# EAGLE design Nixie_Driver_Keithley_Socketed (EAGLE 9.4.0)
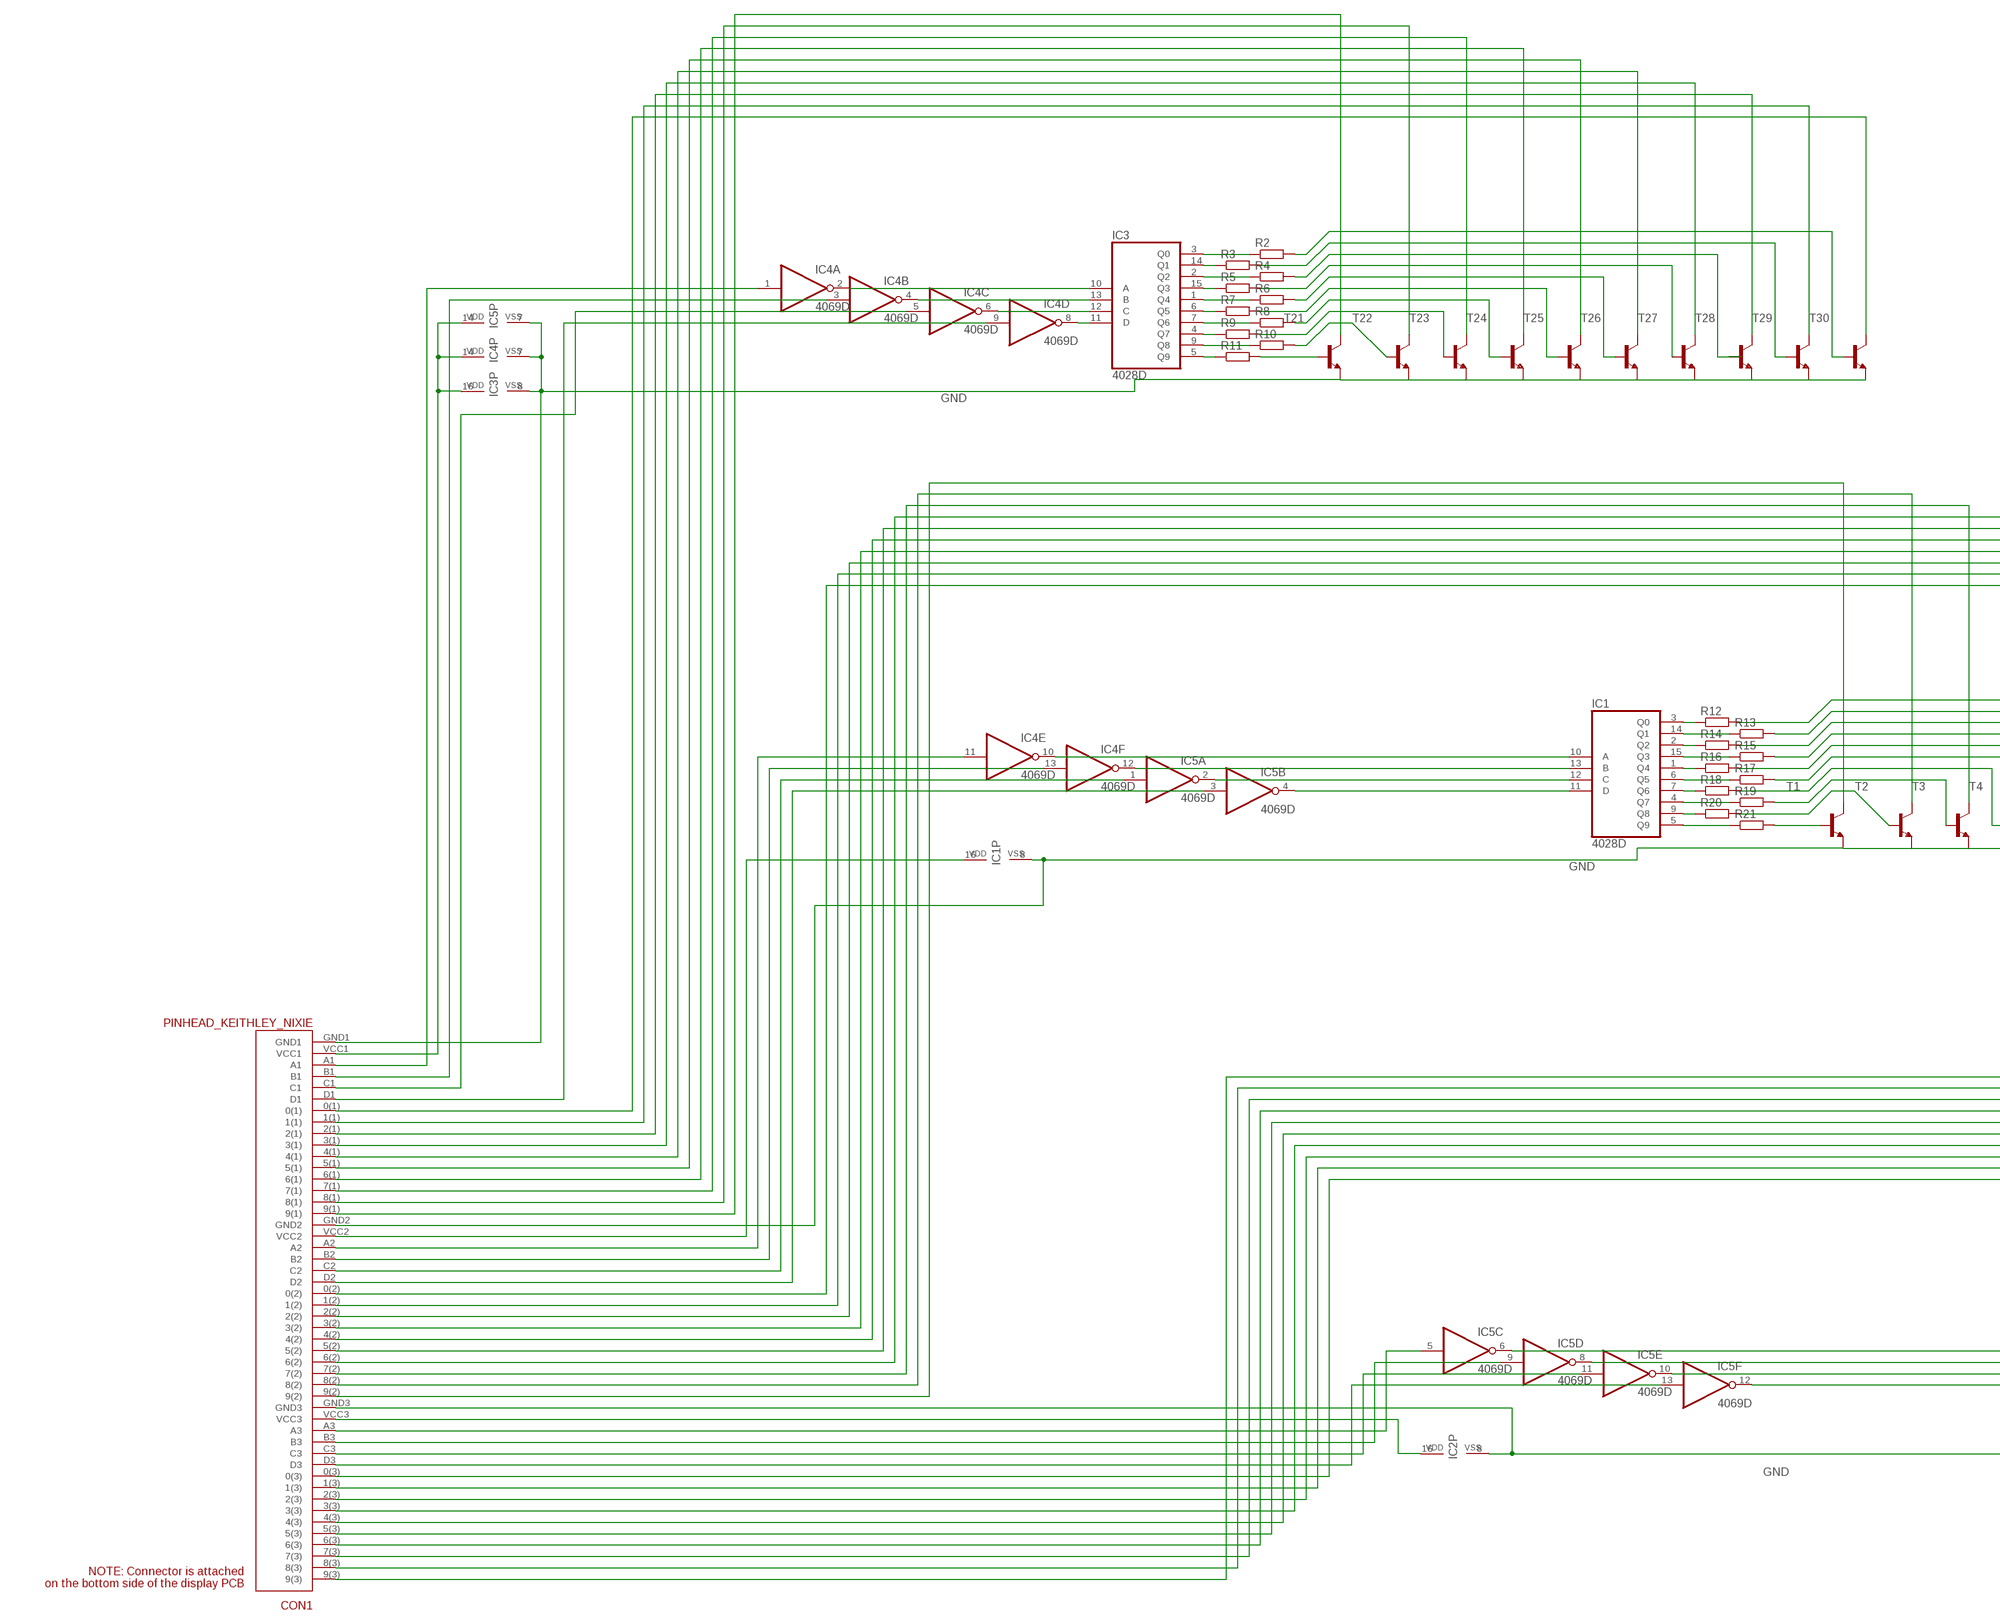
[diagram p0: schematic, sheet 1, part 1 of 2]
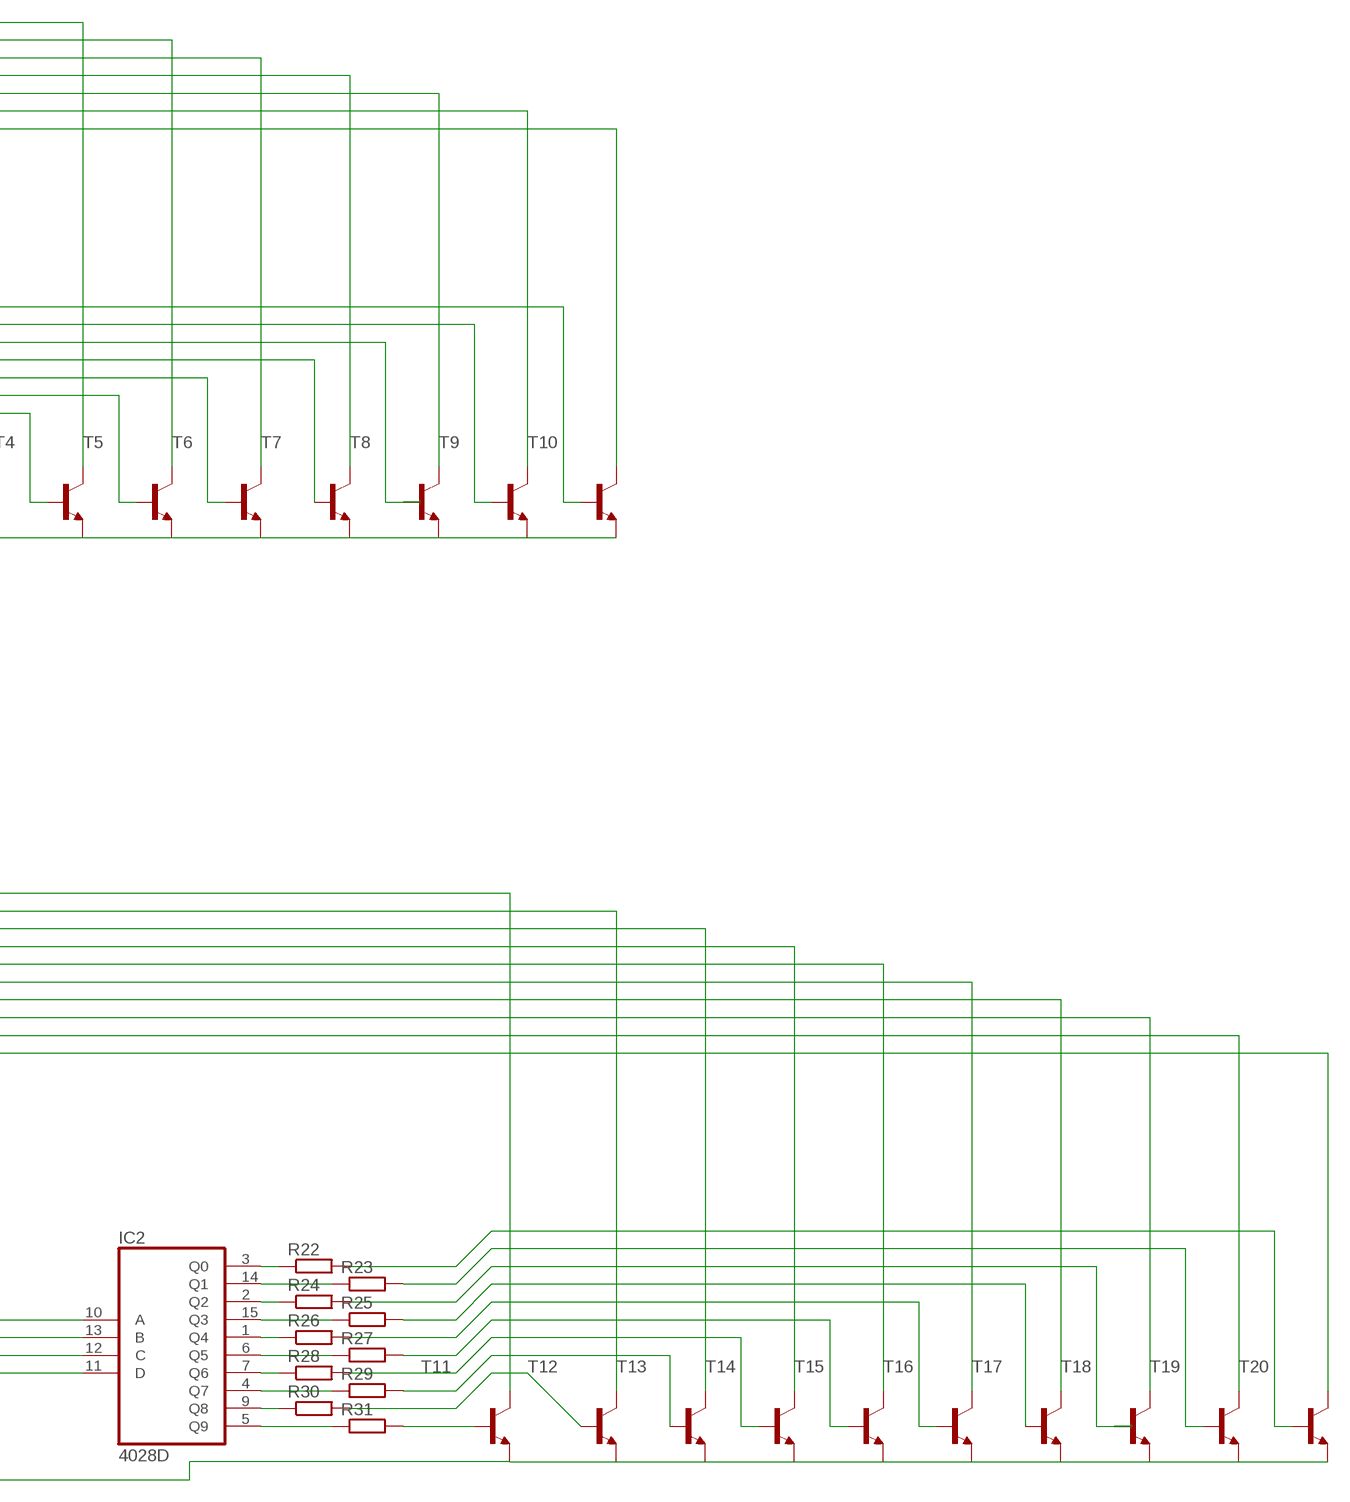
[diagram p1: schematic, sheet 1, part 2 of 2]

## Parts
CON1  PINHEAD_KEITHLEY_NIXIE  [PINHEAD_KEITHLEY_NIXIE]
IC1  4028D  [SO16]
IC2  4028D  [SO16]
IC3  4028D  [SO16]
IC4  4069D  [SO14]
IC5  4069D  [SO14]
R2  R-EU_R0402  [R0402]
R3  R-EU_R0402  [R0402]
R4  R-EU_R0402  [R0402]
R5  R-EU_R0402  [R0402]
R6  R-EU_R0402  [R0402]
R7  R-EU_R0402  [R0402]
R8  R-EU_R0402  [R0402]
R9  R-EU_R0402  [R0402]
R10  R-EU_R0402  [R0402]
R11  R-EU_R0402  [R0402]
R12  R-EU_R0402  [R0402]
R13  R-EU_R0402  [R0402]
R14  R-EU_R0402  [R0402]
R15  R-EU_R0402  [R0402]
R16  R-EU_R0402  [R0402]
R17  R-EU_R0402  [R0402]
R18  R-EU_R0402  [R0402]
R19  R-EU_R0402  [R0402]
R20  R-EU_R0402  [R0402]
R21  R-EU_R0402  [R0402]
R22  R-EU_R0402  [R0402]
R23  R-EU_R0402  [R0402]
R24  R-EU_R0402  [R0402]
R25  R-EU_R0402  [R0402]
R26  R-EU_R0402  [R0402]
R27  R-EU_R0402  [R0402]
R28  R-EU_R0402  [R0402]
R29  R-EU_R0402  [R0402]
R30  R-EU_R0402  [R0402]
R31  R-EU_R0402  [R0402]
T1  MMBTA42LT1-NPN-SOT23-BEC  [SOT23-BEC]
T2  MMBTA42LT1-NPN-SOT23-BEC  [SOT23-BEC]
T3  MMBTA42LT1-NPN-SOT23-BEC  [SOT23-BEC]
T4  MMBTA42LT1-NPN-SOT23-BEC  [SOT23-BEC]
T5  MMBTA42LT1-NPN-SOT23-BEC  [SOT23-BEC]
T6  MMBTA42LT1-NPN-SOT23-BEC  [SOT23-BEC]
T7  MMBTA42LT1-NPN-SOT23-BEC  [SOT23-BEC]
T8  MMBTA42LT1-NPN-SOT23-BEC  [SOT23-BEC]
T9  MMBTA42LT1-NPN-SOT23-BEC  [SOT23-BEC]
T10  MMBTA42LT1-NPN-SOT23-BEC  [SOT23-BEC]
T11  MMBTA42LT1-NPN-SOT23-BEC  [SOT23-BEC]
T12  MMBTA42LT1-NPN-SOT23-BEC  [SOT23-BEC]
T13  MMBTA42LT1-NPN-SOT23-BEC  [SOT23-BEC]
T14  MMBTA42LT1-NPN-SOT23-BEC  [SOT23-BEC]
T15  MMBTA42LT1-NPN-SOT23-BEC  [SOT23-BEC]
T16  MMBTA42LT1-NPN-SOT23-BEC  [SOT23-BEC]
T17  MMBTA42LT1-NPN-SOT23-BEC  [SOT23-BEC]
T18  MMBTA42LT1-NPN-SOT23-BEC  [SOT23-BEC]
T19  MMBTA42LT1-NPN-SOT23-BEC  [SOT23-BEC]
T20  MMBTA42LT1-NPN-SOT23-BEC  [SOT23-BEC]
T21  MMBTA42LT1-NPN-SOT23-BEC  [SOT23-BEC]
T22  MMBTA42LT1-NPN-SOT23-BEC  [SOT23-BEC]
T23  MMBTA42LT1-NPN-SOT23-BEC  [SOT23-BEC]
T24  MMBTA42LT1-NPN-SOT23-BEC  [SOT23-BEC]
T25  MMBTA42LT1-NPN-SOT23-BEC  [SOT23-BEC]
T26  MMBTA42LT1-NPN-SOT23-BEC  [SOT23-BEC]
T27  MMBTA42LT1-NPN-SOT23-BEC  [SOT23-BEC]
T28  MMBTA42LT1-NPN-SOT23-BEC  [SOT23-BEC]
T29  MMBTA42LT1-NPN-SOT23-BEC  [SOT23-BEC]
T30  MMBTA42LT1-NPN-SOT23-BEC  [SOT23-BEC]

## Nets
GND: CON1.GND1 CON1.GND2 CON1.GND3 IC1.8(VSS) IC2.8(VSS) IC3.8(VSS) IC4.7(P:VSS) IC5.7(P:VSS) T1.E T2.E T3.E T4.E T5.E T6.E T7.E T8.E T9.E T10.E T11.E T12.E T13.E T14.E T15.E T16.E T17.E T18.E T19.E T20.E T21.E T22.E T23.E T24.E T25.E T26.E T27.E T28.E T29.E T30.E
N$1: IC1.5(Q9) R21.1
N$2: R20.2 T2.B
N$3: R19.2 T3.B
N$4: R18.2 T4.B
N$5: R17.2 T5.B
N$6: R16.2 T6.B
N$7: R15.2 T7.B
N$8: R14.2 T8.B
N$9: R13.2 T9.B
N$10: R12.2 T10.B
N$11: IC3.10(A) IC4.2(A:O)
N$12 [HV_Cathodes]: CON1.9(2) T1.C
N$13 [HV_Cathodes]: CON1.7(2) T3.C
N$14 [HV_Cathodes]: CON1.5(2) T5.C
N$15 [HV_Cathodes]: CON1.3(2) T7.C
N$16 [HV_Cathodes]: CON1.1(2) T9.C
N$17 [HV_Cathodes]: CON1.8(2) T2.C
N$18: CON1.A2 IC4.11(E:I)
N$19 [HV_Cathodes]: CON1.0(2) T10.C
N$20 [HV_Cathodes]: CON1.2(2) T8.C
N$21 [HV_Cathodes]: CON1.4(2) T6.C
N$22 [HV_Cathodes]: CON1.6(2) T4.C
N$23 [HV_Cathodes]: CON1.8(1) T22.C
N$24: CON1.B2 IC4.13(F:I)
N$25: CON1.VCC2 IC1.16(VDD)
N$26: CON1.C2 IC5.1(A:I)
N$27 [HV_Cathodes]: CON1.8(3) T12.C
N$28: R31.2 T11.B
N$29: R30.2 T12.B
N$30: R29.2 T13.B
N$31: R28.2 T14.B
N$32: R27.2 T15.B
N$33: R26.2 T16.B
N$34: R25.2 T17.B
N$35: R24.2 T18.B
N$36: R23.2 T19.B
N$37: R22.2 T20.B
N$38: IC3.13(B) IC4.4(B:O)
N$39 [HV_Cathodes]: CON1.9(3) T11.C
N$40 [HV_Cathodes]: CON1.7(3) T13.C
N$41 [HV_Cathodes]: CON1.5(3) T15.C
N$42 [HV_Cathodes]: CON1.3(3) T17.C
N$43 [HV_Cathodes]: CON1.1(3) T19.C
N$44: CON1.D2 IC5.3(B:I)
N$45: CON1.A3 IC5.5(C:I)
N$46 [HV_Cathodes]: CON1.0(3) T20.C
N$47 [HV_Cathodes]: CON1.2(3) T18.C
N$48 [HV_Cathodes]: CON1.4(3) T16.C
N$49 [HV_Cathodes]: CON1.6(3) T14.C
N$50: IC3.12(C) IC4.6(C:O)
N$51: CON1.B3 IC5.9(D:I)
N$52: CON1.VCC3 IC2.16(VDD)
N$53: CON1.VCC1 IC3.16(VDD) IC4.14(P:VDD) IC5.14(P:VDD)
N$54: CON1.C3 IC5.11(E:I)
N$55: IC3.11(D) IC4.8(D:O)
N$56: CON1.C1 IC4.5(C:I)
N$57: CON1.D3 IC5.13(F:I)
N$58: IC1.10(A) IC4.10(E:O)
N$59: IC1.13(B) IC4.12(F:O)
N$60: IC1.12(C) IC5.2(A:O)
N$61: IC1.11(D) IC5.4(B:O)
N$62: IC2.10(A) IC5.6(C:O)
N$63: IC2.13(B) IC5.8(D:O)
N$64: IC2.12(C) IC5.10(E:O)
N$65: IC2.11(D) IC5.12(F:O)
N$66: IC3.3(Q0) R2.1
N$67: IC3.14(Q1) R3.1
N$68: IC3.2(Q2) R4.1
N$69: IC3.15(Q3) R5.1
N$70: IC3.1(Q4) R6.1
N$71: IC3.6(Q5) R7.1
N$72: IC3.7(Q6) R8.1
N$73: IC3.4(Q7) R9.1
N$74: IC3.9(Q8) R10.1
N$75: IC3.5(Q9) R11.1
N$76: IC1.3(Q0) R12.1
N$77: IC1.14(Q1) R13.1
N$78: IC1.2(Q2) R14.1
N$79: IC1.15(Q3) R15.1
N$80: IC1.1(Q4) R16.1
N$81: IC1.6(Q5) R17.1
N$82: IC1.7(Q6) R18.1
N$83: IC1.4(Q7) R19.1
N$84: IC1.9(Q8) R20.1
N$85: R11.2 T21.B
N$86: R10.2 T22.B
N$87: R9.2 T23.B
N$88: R8.2 T24.B
N$89: R7.2 T25.B
N$90: R6.2 T26.B
N$91: R5.2 T27.B
N$92: R4.2 T28.B
N$93: R3.2 T29.B
N$94: R2.2 T30.B
N$95: R21.2 T1.B
N$96 [HV_Cathodes]: CON1.9(1) T21.C
N$97 [HV_Cathodes]: CON1.7(1) T23.C
N$98 [HV_Cathodes]: CON1.5(1) T25.C
N$99 [HV_Cathodes]: CON1.3(1) T27.C
N$100 [HV_Cathodes]: CON1.1(1) T29.C
N$101: CON1.A1 IC4.1(A:I)
N$102: CON1.B1 IC4.3(B:I)
N$103: IC2.3(Q0) R22.1
N$104 [HV_Cathodes]: CON1.0(1) T30.C
N$105 [HV_Cathodes]: CON1.2(1) T28.C
N$106 [HV_Cathodes]: CON1.4(1) T26.C
N$107 [HV_Cathodes]: CON1.6(1) T24.C
N$108: IC2.14(Q1) R23.1
N$109: CON1.D1 IC4.9(D:I)
N$110: IC2.2(Q2) R24.1
N$111: IC2.15(Q3) R25.1
N$112: IC2.1(Q4) R26.1
N$113: IC2.6(Q5) R27.1
N$114: IC2.7(Q6) R28.1
N$115: IC2.4(Q7) R29.1
N$116: IC2.9(Q8) R30.1
N$117: IC2.5(Q9) R31.1

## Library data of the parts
CON1 = DIL_Style_Pinhead_Connectors:PINHEAD_KEITHLEY_NIXIE
IC1-IC3 = 40xx:4028: BCD to decimal DECODER
IC4 IC5 = 40xx:4069: Hex INVERTER
R2-R31 = rcl:R-EU_: RESISTOR, European symbol; SPICEPREFIX: R
T1-T30 = transistor-neu-to92:*-NPN-: NPN Transistror

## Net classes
0 LV_Signal: width 0.25 mm, clearance 0.3 mm
1 HV_Cathodes: width 0.25 mm, clearance 0.6 mm

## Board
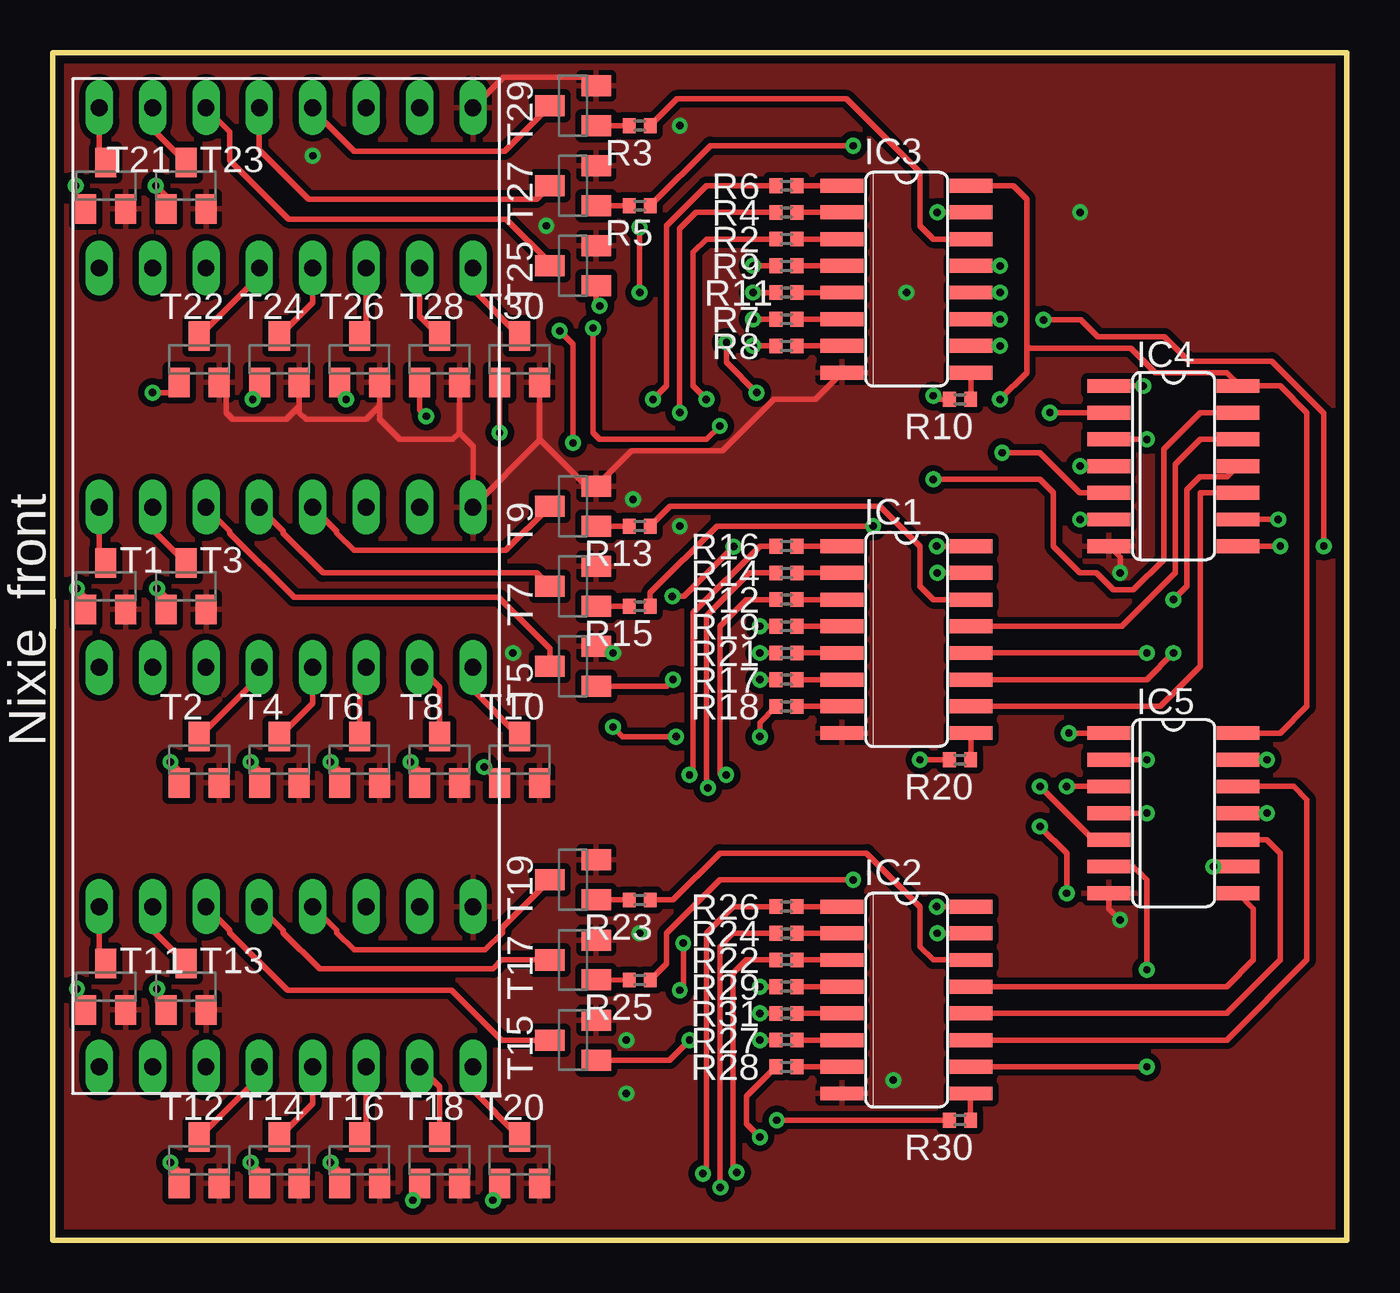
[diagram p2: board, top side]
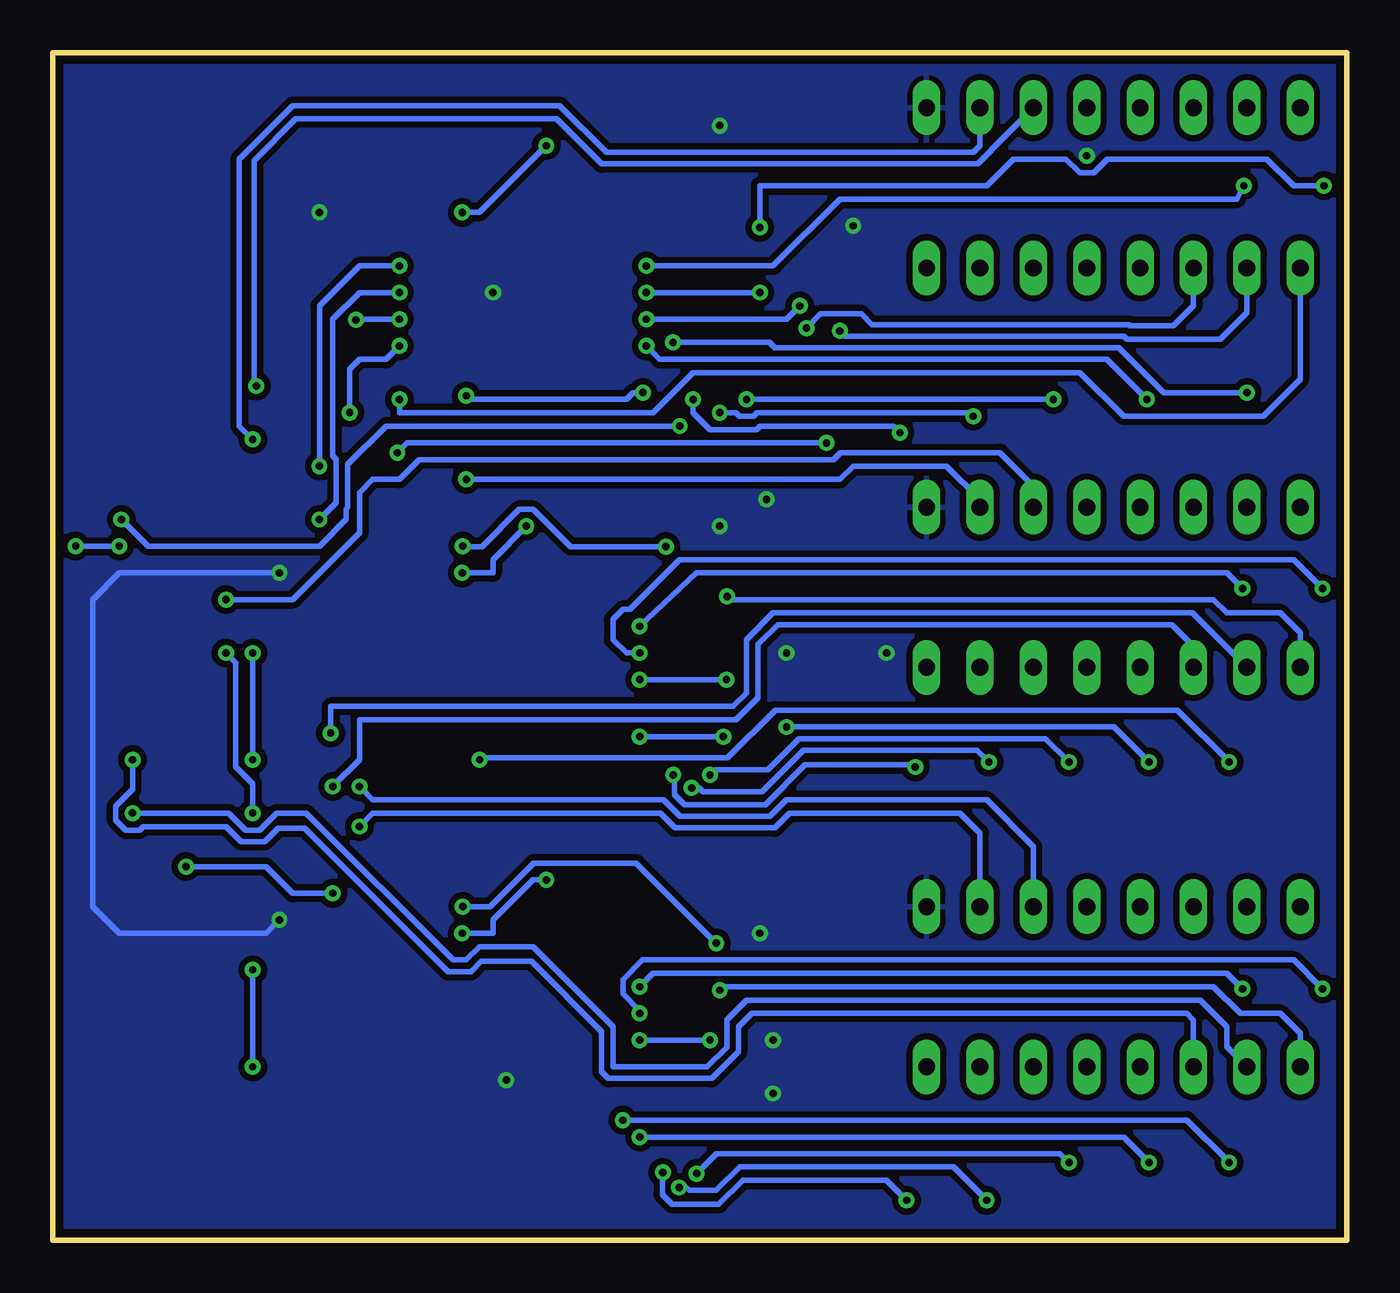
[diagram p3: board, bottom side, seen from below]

Size 61.59 x 56.5 mm. Coordinates in mm from the lower left corner, seen from the top.
Outline: 0,0 61.59,0 61.59,56.5 0,56.5 0,0
Copper layers (1*16): Top 0.035mm / dielectric 1.5mm / Bottom 0.035mm
Design rules "default *": minimum track width 0.25mm, minimum drill 0.35mm, track to track 0.3mm, track to pad 0.3mm, pad to pad 0.3mm, via to via 0.3mm, smd to smd 0mil, copper to edge 0.4mm, drill to drill 6mil, minimum pad ring 10mil, minimum via ring 8mil, stop-mask expansion 4mil, vias tented up to drill 0mil, thermal gap 10mil

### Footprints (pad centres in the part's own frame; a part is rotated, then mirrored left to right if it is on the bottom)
PINHEAD_KEITHLEY_NIXIE = drill 0.8 long: 0(1) 38,-17.78; 0(2) 19,-17.78; 0(3) 0,-17.78; 1(1) 45.62,-10.16; 1(2) 26.62,-10.16; 1(3) 7.62,-10.16; 2(1) 38,-15.24; 2(2) 19,-15.24; 2(3) 0,-15.24; 3(1) 45.62,-7.62; 3(2) 26.62,-7.62; 3(3) 7.62,-7.62; 4(1) 38,-12.7; 4(2) 19,-12.7; 4(3) 0,-12.7; 5(1) 45.62,-5.08; 5(2) 26.62,-5.08; 5(3) 7.62,-5.08; 6(1) 38,-10.16; 6(2) 19,-10.16; 6(3) 0,-10.16; 7(1) 45.62,-2.54; 7(2) 26.62,-2.54; 7(3) 7.62,-2.54; 8(1) 38,-7.62; 8(2) 19,-7.62; 8(3) 0,-7.62; 9(1) 45.62,0; 9(2) 26.62,0; 9(3) 7.62,0; A1 45.62,-12.7; A2 26.62,-12.7; A3 7.62,-12.7; B1 45.62,-15.24; B2 26.62,-15.24; B3 7.62,-15.24; C1 38,-2.54; C2 19,-2.54; C3 0,-2.54; D1 38,-5.08; D2 19,-5.08; D3 0,-5.08; GND1 45.62,-17.78; GND2 26.62,-17.78; GND3 7.62,-17.78; VCC1 38,0; VCC2 19,0; VCC3 0,0
SO16 = smd 0.66 x 2.032: 1 -4.445,-3.073; 2 -3.175,-3.073; 3 -1.905,-3.073; 4 -0.635,-3.073; 5 0.635,-3.073; 6 1.905,-3.073; 7 3.175,-3.073; 8 4.445,-3.073; 9 4.445,3.073; 10 3.175,3.073; 11 1.905,3.073; 12 0.635,3.073; 13 -0.635,3.073; 14 -1.905,3.073; 15 -3.175,3.073; 16 -4.445,3.073
SO14 = smd 0.66 x 2.032: 1 -3.81,-3.073; 2 -2.54,-3.073; 3 -1.27,-3.073; 4 0,-3.073; 5 1.27,-3.073; 6 2.54,-3.073; 7 3.81,-3.073; 8 3.81,3.073; 9 2.54,3.073; 10 1.27,3.073; 11 0,3.073; 12 -1.27,3.073; 13 -2.54,3.073; 14 -3.81,3.073
R0402 = smd 0.6 x 0.7: 1 -0.5,0; 2 0.5,0
SOT23-BEC = smd 1 x 1.4: B -0.95,-1.1; C 0,1.1; E 0.95,-1.1

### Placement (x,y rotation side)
CON1  2.22,8.26 90 top
IC1  40.64,28.57 270 top
IC2  40.64,11.43 270 top
IC3  40.64,45.72 270 top
IC4  53.34,36.83 270 top
IC5  53.34,20.32 270 top
R2  34.92,47.62 180 top
R3  27.94,53.02 180 top
R4  34.92,48.9 180 top
R5  27.94,49.21 180 top
R6  34.92,50.16 180 top
R7  34.92,43.81 180 top
R8  34.92,42.55 180 top
R9  34.92,46.35 180 top
R10  43.18,40.01 180 top
R11  34.92,45.09 180 top
R12  34.92,30.48 180 top
R13  27.94,33.97 180 top
R14  34.92,31.75 180 top
R15  27.94,30.16 180 top
R16  34.92,33.02 180 top
R17  34.92,26.67 180 top
R18  34.92,25.4 180 top
R19  34.92,29.21 180 top
R20  43.18,22.86 180 top
R21  34.92,27.94 180 top
R22  34.92,13.34 180 top
R23  27.94,16.19 180 top
R24  34.92,14.61 180 top
R25  27.94,12.38 180 top
R26  34.92,15.88 180 top
R27  34.92,9.53 180 top
R28  34.92,8.26 180 top
R29  34.92,12.06 180 top
R30  43.18,5.71 180 top
R31  34.92,10.79 180 top
T1  2.54,31.11 0 top
T2  6.99,22.86 0 top
T3  6.35,31.11 0 top
T4  10.79,22.86 0 top
T5  24.77,27.3 90 top
T6  14.61,22.86 0 top
T7  24.77,31.11 90 top
T8  18.41,22.86 0 top
T9  24.77,34.92 90 top
T10  22.23,22.86 0 top
T11  2.54,12.06 0 top
T12  6.99,3.81 0 top
T13  6.35,12.06 0 top
T14  10.79,3.81 0 top
T15  24.77,9.53 90 top
T16  14.61,3.81 0 top
T17  24.77,13.34 90 top
T18  18.41,3.81 0 top
T19  24.77,17.14 90 top
T20  22.23,3.81 0 top
T21  2.54,50.16 0 top
T22  6.99,41.91 0 top
T23  6.35,50.16 0 top
T24  10.79,41.91 0 top
T25  24.77,46.35 90 top
T26  14.61,41.91 0 top
T27  24.77,50.16 90 top
T28  18.41,41.91 0 top
T29  24.77,53.98 90 top
T30  22.23,41.91 0 top

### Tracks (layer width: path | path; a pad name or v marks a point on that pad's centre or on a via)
GND  (via drill 0.35)
  Top 0.25: CON1.GND1 21.46,55.33 25.46,55.33 T29.E | T22.E 8.26,40.49 8.26,39.37 8.57,39.05 11.11,39.05 11.74,39.69 | T24.E 11.74,39.69 | T26.E 15.55,39.69 | 15.55,39.69 15.56,39.69 14.92,39.05 12.06,39.05 11.74,39.37 11.74,39.69 | T30.E 23.18,38.1 | 23.18,38.1 23.18,38.05 CON1.GND2 20,37.78 19.36,38.42 | T28.E 19.36,38.42 | 15.55,39.69 15.55,39.05 16.51,38.1 19.05,38.1 19.36,38.42 | IC4.7 50.8,32.49 v50.8,31.75 | v50.8,15.24 50.27,15.77 IC5.7 | IC3.8 36.3,40.01 34.32,40.01 31.87,37.55 27.54,37.55 T9.E 25.4,35.88 23.18,38.1
  Bottom 0.25: v50.8,31.75 58.42,31.75 59.69,30.48 59.69,15.88 58.42,14.61 51.44,14.61 v50.8,15.24
  other vias: 12.38,51.59 40.01,7.62 27.3,9.53 27.3,6.99 27.94,14.61 29.84,53.02 40.64,45.09 48.9,48.9 29.84,33.97 27.62,35.24 23.5,48.26 21.91,27.94 26.67,27.94
  pour Top: 0,56.52 61.59,56.52 61.59,0 0,0
  pour Bottom: 0,56.52 61.59,56.52 61.59,0 0,0
N$1
  Top 0.25: R21.1 IC1.5
N$2  (via drill 0.35)
  Top 0.25: R20.2 v41.27,22.86 | v5.61,22.75 6.04,22.33 T2.B
  Bottom 0.25: v41.27,22.86 41.19,22.95 29.47,22.95 27.2,25.22 8.08,25.22 v5.61,22.75
N$3  (via drill 0.35)
  Top 0.25: T3.B 5.4,30.58 v4.97,31.01 | R19.2 v33.66,29.21
  Bottom 0.25: v4.97,31.01 5.71,31.75 30.95,31.75 v33.66,29.21
N$4  (via drill 0.35)
  Top 0.25: R18.2 33.66,24.63 v33.66,23.96 | v29.68,23.96 27.13,23.96 v26.67,24.42 | v9.42,22.75 9.85,22.33 T4.B
  Bottom 0.25: v33.66,23.96 v29.68,23.96 | v26.67,24.42 11.08,24.42 v9.42,22.75
N$5  (via drill 0.35)
  Top 0.25: R17.2 v33.66,26.67 | v29.53,26.67 29.21,26.36 T5.B
  Bottom 0.25: v33.66,26.67 v29.53,26.67
N$6  (via drill 0.35)
  Top 0.25: R16.2 33.66,33.02 30.48,29.84 30.48,22.23 30.4,22.14 v30.31,22.14 | v13.23,22.75 13.65,22.33 T6.B
  Bottom 0.25: v30.31,22.14 30.06,22.39 27.56,22.39 26.08,23.87 14.34,23.87 v13.23,22.75
N$7
  Top 0.25: T7.B R15.2
N$8  (via drill 0.35)
  Top 0.25: R14.2 33.16,31.75 31.11,29.7 31.11,21.59 v31.18,21.52 | v17.04,22.75 17.46,22.33 T8.B
  Bottom 0.25: v31.18,21.52 30.83,21.52 30.64,21.34 27.84,21.34 25.86,23.32 17.6,23.32 v17.04,22.75
N$9
  Top 0.25: T9.B R13.2
N$10  (via drill 0.35)
  Top 0.25: R12.2 33.02,30.48 31.75,29.21 31.75,22.23 31.83,22.14 v32.06,22.14 | v20.54,22.51 21.27,21.78 T10.B
  Bottom 0.25: v32.06,22.14 31.99,22.07 31.99,21.19 31.52,20.72 27.68,20.72 25.79,22.61 20.64,22.61 v20.54,22.51
N$11  (via drill 0.35)
  Top 0.25: IC3.10 v45.09,42.55 | v47.46,39.37 IC4.2
  Bottom 0.25: v45.09,42.55 45.72,41.91 46.99,41.91 47.46,41.44 v47.46,39.37
N$12
  Top 0.25: T1.C 2.22,32.53 CON1.9(2)
N$13
  Top 0.25: T3.C 4.76,33.8 CON1.7(2)
N$14
  Top 0.25: CON1.5(2) 8.44,33.74 8.44,33.64 11.49,30.58 21.22,30.58 23.66,28.14 T5.C
N$15
  Top 0.25: CON1.3(2) 10.98,33.74 10.98,33.64 12.87,31.75 23.03,31.75 T7.C
N$16
  Top 0.25: CON1.1(2) 13.52,33.74 13.52,33.64 14.34,32.82 21.56,32.82 T9.C
N$17
  Top 0.25: T2.C 9.84,26.82 CON1.8(2)
N$18  (via drill 0.35)
  Top 0.25: IC4.11 55.9,36.31 54.59,36.31 53.98,35.7 53.98,31.11 v53.34,30.48
  Bottom 0.25: v53.34,30.48 50.16,30.48 46.99,33.66 46.99,35.56 46.35,36.2 45.09,36.2 44.15,37.13 24.43,37.13 24.1,37.47 16.51,37.47 14.92,35.88 CON1.A2
N$19
  Top 0.25: T10.C 20,26.18 CON1.0(2)
N$20
  Top 0.25: T8.C 18.41,26.3 CON1.2(2)
N$21
  Top 0.25: T6.C 14.61,26.94 CON1.4(2)
N$22
  Top 0.25: T4.C 12.38,25.55 CON1.6(2)
N$23
  Top 0.25: T22.C 9.84,45.87 CON1.8(1)
N$24  (via drill 0.35)
  Top 0.25: IC4.13 54.61,39.37 52.88,37.63 52.88,32.38 51.44,30.95 50.47,30.95 49.66,31.75 48.9,31.75 47.62,33.02 47.62,35.56 46.99,36.2 v41.91,36.2
  Bottom 0.25: v41.91,36.2 24.13,36.2 23.5,36.83 19.05,36.83 17.46,35.24 CON1.B2
N$25  (via drill 0.35)
  Top 0.25: v32.41,33 30.04,30.63 v29.49,30.63 | v42.08,33.02 IC1.16
  Bottom 0.25: CON1.VCC2 2.22,28.89 3.17,29.84 5.71,29.84 6.35,30.48 29.3,30.48 v29.49,30.63 | v42.08,33.02 42.05,33 41.16,33 39.38,34.78 38.72,34.78 36.94,33 v32.41,33
N$26  (via drill 0.35)
  Top 0.25: v48.36,24.13 IC5.1
  Bottom 0.25: CON1.C2 7.35,29.84 27.3,29.84 28.57,28.57 28.57,26.04 29.21,25.4 48.36,25.4 v48.36,24.13
N$27
  Top 0.25: T12.C 9.84,7.77 CON1.8(3)
N$28  (via drill 0.35)
  Top 0.25: T11.B 1.16,11.39 v1.16,11.96 | v33.66,10.79 R31.2
  Bottom 0.25: v1.16,11.96 2.54,13.34 33.52,13.34 34.46,12.4 34.46,11.73 33.66,10.93 v33.66,10.79
N$29  (via drill 0.35)
  Top 0.25: R30.2 v34.46,5.71 | v5.61,3.7 6.04,3.28 T12.B
  Bottom 0.25: v34.46,5.71 7.62,5.71 v5.61,3.7
N$30  (via drill 0.35)
  Top 0.25: T13.B 4.97,11.39 v4.97,11.96 | v33.66,12.06 R29.2
  Bottom 0.25: v4.97,11.96 5.71,12.7 33.02,12.7 v33.66,12.06
N$31  (via drill 0.35)
  Top 0.25: R28.2 33.02,6.85 33.02,5.55 v33.66,4.91 | v9.42,3.7 9.85,3.28 T14.B
  Bottom 0.25: v33.66,4.91 10.63,4.91 v9.42,3.7
N$32  (via drill 0.35)
  Top 0.25: R27.2 v33.66,9.53 | v30.31,9.53 29.36,8.57 T15.B
  Bottom 0.25: v33.66,9.53 v30.31,9.53
N$33  (via drill 0.35)
  Top 0.25: R26.2 32.38,15.88 31.11,14.61 31.11,3.17 v30.95,3.17 | v13.23,3.7 13.65,3.28 T16.B
  Bottom 0.25: v30.95,3.17 29.99,4.13 13.65,4.13 v13.23,3.7
N$34
  Top 0.25: T17.B R25.2
N$35  (via drill 0.35)
  Top 0.25: R24.2 32.38,14.61 31.75,13.97 31.75,2.54 v31.78,2.51 | T18.B 17.46,2.23 v17.14,1.91
  Bottom 0.25: v31.78,2.51 31.42,2.51 31.28,2.37 30.01,2.37 28.89,3.49 18.73,3.49 v17.14,1.91
N$36
  Top 0.25: T19.B R23.2 arc-90 R23.2
N$37  (via drill 0.35)
  Top 0.25: R22.2 33.02,13.34 32.38,12.7 32.38,3.17 32.44,3.23 v32.55,3.23 | v20.95,1.91 21.27,2.23 T20.B
  Bottom 0.25: v32.55,3.23 32.55,2.87 32.58,2.85 32.58,2.18 32.11,1.71 29.9,1.71 28.75,2.86 21.91,2.86 v20.95,1.91
N$38  (via drill 0.35)
  Top 0.25: IC3.13 v45.09,46.35 | v48.9,36.83 IC4.4
  Bottom 0.25: v45.09,46.35 46.99,46.35 48.9,44.45 v48.9,36.83
N$39
  Top 0.25: CON1.9(3) 2.22,13.48 T11.C
N$40
  Top 0.25: CON1.7(3) 4.76,14.75 T13.C
N$41
  Top 0.25: T15.C 21.37,9.53 19,11.9 11.18,11.9 8.44,14.64 8.44,14.74 CON1.5(3)
N$42
  Top 0.25: T17.C 21.38,13.34 20.96,12.92 12.7,12.92 10.98,14.64 10.98,14.74 CON1.3(3)
N$43
  Top 0.25: CON1.1(3) 13.52,14.74 13.52,14.64 14.34,13.82 20.58,13.82 21.41,14.64 21.41,14.89 T19.C
N$44  (via drill 0.35)
  Top 0.25: v48.26,21.59 IC5.3
  Bottom 0.25: CON1.D2 7.3,28.26 8.33,29.29 27.08,29.29 28.02,28.35 28.02,25.81 29.07,24.77 46.99,24.77 46.99,22.86 v48.26,21.59
N$45  (via drill 0.35)
  Top 0.25: v46.99,21.59 49.53,19.05 IC5.5
  Bottom 0.25: CON1.A3 14.92,18.73 17.14,20.95 26.66,20.95 27.45,20.17 31.75,20.17 32.53,20.95 46.35,20.95 v46.99,21.59
N$46
  Top 0.25: CON1.0(3) 20,7.13 T20.C
N$47
  Top 0.25: T18.C 18.41,7.3 CON1.2(3)
N$48
  Top 0.25: T16.C 14.92,5.23 CON1.4(3)
N$49
  Top 0.25: T14.C 12.38,6.5 CON1.6(3)
N$50  (via drill 0.35)
  Top 0.25: IC3.12 v45.09,45.09 | v48.9,34.29 IC4.6
  Bottom 0.25: v45.09,45.09 46.99,45.09 48.26,43.81 48.26,37.33 48.09,37.16 48.09,35.09 v48.9,34.29
N$51  (via drill 0.35)
  Top 0.25: v46.99,19.68 48.26,18.41 v48.26,16.51 | v55.24,17.78 IC5.9
  Bottom 0.25: CON1.B3 17.46,19.37 18.41,20.32 26.52,20.32 27.22,19.62 31.97,19.62 32.68,20.32 46.35,20.32 v46.99,19.68 | v48.26,16.51 50.16,16.51 51.44,17.78 v55.24,17.78
N$52  (via drill 0.35)
  Top 0.25: v29.84,11.9 30.01,12.06 v30.01,14.14 | v42.08,15.88 IC2.16
  Bottom 0.25: CON1.VCC3 2.22,9.84 3.17,10.79 5.08,10.79 6.35,12.06 29.68,12.06 v29.84,11.9 | v42.08,15.88 40.78,15.88 38.71,17.95 33.82,17.95 v30.01,14.14
N$53  (via drill 0.35)
  Top 0.25: IC4.14 56.52,40.64 | 56.52,40.64 58.42,40.64 59.69,39.37 59.69,25.4 58.42,24.13 IC5.14 | 56.52,40.64 55.88,41.27 52.47,41.27 51.31,42.42 46.48,42.42 46.35,42.55 | v45.09,40.01 46.35,41.27 46.35,42.55 | 46.35,42.55 46.35,49.53 45.72,50.16 IC3.16
  Bottom 0.25: CON1.VCC1 2.22,40.96 3.98,39.2 10.63,39.2 12.7,41.27 31.11,41.27 33.02,39.37 45.09,39.37 v45.09,40.01
N$54  (via drill 0.35)
  Top 0.25: v57.78,20.32 IC5.11
  Bottom 0.25: CON1.C3 5.71,9.21 5.71,10.16 6.99,11.43 28.57,11.43 29.51,10.5 29.51,9.19 30.45,8.26 34.92,8.26 34.92,10.16 38.73,13.97 41.27,13.97 41.91,13.34 42.55,13.34 49.53,20.32 50.93,20.32 51.74,19.52 52.4,19.52 53.21,20.32 v57.78,20.32
N$55  (via drill 0.35)
  Top 0.25: IC3.11 v45.09,43.81 | v47.16,43.78 48.93,43.78 49.73,42.98 52.91,42.98 54.06,41.83 58.01,41.83 60.49,39.34 v60.49,33.02 | v58.42,33.02 IC4.8
  Bottom 0.25: v45.09,43.81 47.12,43.81 v47.16,43.78 | v60.49,33.02 v58.42,33.02
N$56  (via drill 0.35)
  Top 0.25: v24.13,43.26 24.77,42.63 v24.77,37.93 | v45.19,37.47 46.99,37.47 48.9,35.56 IC4.5
  Bottom 0.25: CON1.C1 4.76,44.13 6.03,42.86 10.47,42.86 10.62,43.01 23.88,43.01 v24.13,43.26 | v24.77,37.93 44.72,37.93 v45.19,37.47
N$57  (via drill 0.35)
  Top 0.25: v57.78,22.86 IC5.13
  Bottom 0.25: CON1.D3 7.3,10.48 7.62,10.79 28.32,10.79 28.96,10.16 28.96,8.96 30.22,7.71 35.15,7.71 35.48,8.03 35.48,9.93 38.81,13.26 41.2,13.26 41.68,12.79 42.77,12.79 49.6,19.61 50.86,19.61 51.51,18.97 52.63,18.97 53.34,19.68 57.29,19.68 57.45,19.52 58.12,19.52 58.59,19.99 58.59,20.65 57.78,21.46 v57.78,22.86
N$58
  Top 0.25: IC4.10 54.61,35.56 54.61,27.3 52.7,25.4 IC1.10
N$59
  Top 0.25: IC4.12 54.61,38.1 53.42,36.91 53.42,31.75 50.88,29.21 IC1.13
N$60  (via drill 0.35)
  Top 0.25: IC1.12 v52.07,27.94 | v52.07,22.86 IC5.2
  Bottom 0.25: v52.07,27.94 v52.07,22.86
N$61  (via drill 0.35)
  Top 0.25: IC1.11 52.07,26.67 v53.34,27.94 | v52.07,20.32 IC5.4
  Bottom 0.25: v52.07,20.32 52.07,21.72 52.87,22.53 52.87,27.47 v53.34,27.94
N$62  (via drill 0.35)
  Top 0.25: IC5.6 51.44,17.78 52.07,17.14 v52.07,12.87 | v52.07,8.26 IC2.10
  Bottom 0.25: v52.07,12.87 v52.07,8.26
N$63
  Top 0.25: IC5.8 57.15,15.77 57.15,13.34 55.88,12.06 IC2.13
N$64
  Top 0.25: IC5.10 57.78,19.05 58.42,18.41 58.42,13.34 55.88,10.79 IC2.12
N$65
  Top 0.25: IC5.12 59.05,21.59 59.69,20.95 59.69,13.34 55.88,9.53 IC2.11
N$66
  Top 0.25: R2.1 IC3.3
N$67
  Top 0.25: R3.1 29.71,54.29 37.78,54.29 41.27,50.8 41.27,48.26 41.91,47.62 IC3.14
N$68
  Top 0.25: R4.1 IC3.2
N$69  (via drill 0.35)
  Top 0.25: R5.1 31.3,52.07 v38.1,52.07 | v42.1,48.9 IC3.15
  Bottom 0.25: v38.1,52.07 41.27,48.9 v42.1,48.9
N$70
  Top 0.25: R6.1 IC3.1
N$71
  Top 0.25: R7.1 IC3.6
N$72
  Top 0.25: R8.1 IC3.7
N$73
  Top 0.25: R9.1 IC3.4
N$74
  Top 0.25: R10.1 IC3.9
N$75
  Top 0.25: R11.1 IC3.5
N$76
  Top 0.25: R12.1 IC1.3
N$77
  Top 0.25: R13.1 29.39,34.92 39.37,34.92 41.27,33.02 41.27,31.11 41.91,30.48 IC1.14
N$78
  Top 0.25: R14.1 IC1.2
N$79  (via drill 0.35)
  Top 0.25: R15.1 28.44,30.8 31.61,33.97 v39.05,33.97 | v42.1,31.75 IC1.15
  Bottom 0.25: v39.05,33.97 40.64,32.38 40.64,31.75 v42.1,31.75
N$80
  Top 0.25: R16.1 IC1.1
N$81
  Top 0.25: R17.1 IC1.6
N$82
  Top 0.25: R18.1 IC1.7
N$83
  Top 0.25: R19.1 IC1.4
N$84
  Top 0.25: R20.1 IC1.9
N$85  (via drill 0.35)
  Top 0.25: R11.2 v33.34,45.09 | v1.1,50.16 1.1,49.56 T21.B | v27.94,45.09 v27.94,48.18
  Bottom 0.25: v33.34,45.09 v27.94,45.09 | v1.1,50.16 2.54,50.16 3.81,51.44 11.4,51.44 12.05,50.79 12.71,50.79 13.37,51.44 15.88,51.44 17.14,50.16 27.94,50.16 v27.94,48.18
N$86  (via drill 0.35)
  Top 0.25: v32.07,42.71 32.07,41.76 v33.51,40.32 | v4.76,40.32 5.55,40.32 T22.B | v41.91,40.17 42.08,40.01 R10.2
  Bottom 0.25: v32.07,42.71 27.47,42.71 27.22,42.46 10.84,42.46 8.71,40.32 v4.76,40.32 | v33.51,40.32 33.97,40.32 34.29,40.01 41.74,40.01 v41.91,40.17
N$87  (via drill 0.35)
  Top 0.25: R9.2 v33.34,46.35 | v4.91,50.17 5.4,49.68 T23.B
  Bottom 0.25: v33.34,46.35 27.3,46.35 24.13,49.53 5.23,49.53 v4.91,50.17
N$88  (via drill 0.35)
  Top 0.25: R8.2 v33.34,42.55 | v9.53,40.01 9.85,40.33 T24.B
  Bottom 0.25: v33.34,42.55 32.7,41.91 11.43,41.91 v9.53,40.01
N$89  (via drill 0.35)
  Top 0.25: R7.2 v33.34,43.81 | v26.04,44.45 25.86,44.62 T25.B
  Bottom 0.25: v33.34,43.81 26.67,43.81 v26.04,44.45
N$90  (via drill 0.35)
  Top 0.25: R6.2 31.11,50.16 29.21,48.26 29.21,40.64 v28.57,40.01 | v13.97,40.01 13.97,40.49 T26.B
  Bottom 0.25: v28.57,40.01 v13.97,40.01
N$91
  Top 0.25: T27.B R5.2
N$92  (via drill 0.35)
  Top 0.25: R4.2 30.62,48.9 29.84,48.12 v29.84,39.37 | v17.78,39.2 17.46,39.52 T28.B
  Bottom 0.25: v17.78,39.2 17.95,39.37 28.07,39.37 28.24,39.2 28.91,39.2 29.08,39.37 v29.84,39.37
N$93
  Top 0.25: T29.B R3.2
N$94  (via drill 0.35)
  Top 0.25: R2.2 31.11,47.62 30.48,46.99 30.48,40.64 v31.11,40.01 | v21.27,38.42 T30.B
  Bottom 0.25: v31.11,40.01 31.11,39.37 30.31,38.57 28.1,38.57 27.93,38.73 21.59,38.73 v21.27,38.42
N$95  (via drill 0.35)
  Top 0.25: T1.B 1.59,30.58 v1.16,31.01 | v33.66,27.94 R21.2
  Bottom 0.25: v1.16,31.01 2.54,32.38 31.75,32.38 34.12,30.01 34.45,30.01 34.92,29.54 34.92,28.57 34.29,27.94 v33.66,27.94
N$96
  Top 0.25: CON1.9(1) 2.22,51.58 T21.C
N$97
  Top 0.25: CON1.7(1) 4.76,52.85 T23.C
N$98
  Top 0.25: CON1.5(1) 8.44,52.74 8.44,51.37 11.23,48.58 21.59,48.58 23.66,46.5 T25.C
N$99
  Top 0.25: CON1.3(1) 9.84,51.87 12.18,49.53 23.03,49.53 T27.C
N$100
  Top 0.25: CON1.1(1) 12.38,53.77 14.34,51.82 21.51,51.82 T29.C
N$101  (via drill 0.35)
  Top 0.25: v51.9,40.64 IC4.1
  Bottom 0.25: CON1.A1 16.91,51.88 16.91,51.84 17.55,51.2 35.47,51.2 37.61,53.34 50.02,53.34 52,51.36 52,40.74 v51.9,40.64
N$102  (via drill 0.35)
  Top 0.25: v52.07,38.1 IC4.3
  Bottom 0.25: CON1.B1 17.46,52.07 17.78,51.75 35.24,51.75 37.47,53.98 50.16,53.98 52.7,51.44 52.7,38.73 v52.07,38.1
N$103
  Top 0.25: IC2.3 R22.1
N$104
  Top 0.25: T30.C 20,45.23 CON1.0(1)
N$105
  Top 0.25: T28.C 17.46,43.96 CON1.2(1)
N$106
  Top 0.25: T26.C 14.92,43.33 CON1.4(1)
N$107
  Top 0.25: T24.C 12.38,44.6 CON1.6(1)
N$108
  Top 0.25: R23.1 29.53,16.19 31.75,18.41 38.73,18.41 41.27,15.88 41.27,13.97 41.91,13.34 IC2.14
N$109  (via drill 0.35)
  Top 0.25: v25.72,43.39 25.72,38.42 26.04,38.1 31.11,38.1 v31.75,38.73 | v58.32,34.29 IC4.9
  Bottom 0.25: CON1.D1 7.3,44.45 8.26,43.5 10.33,43.5 10.39,43.56 22.61,43.56 23.11,44.07 25.05,44.07 v25.72,43.39 | v58.32,34.29 57.05,33.02 48.9,33.02 47.62,34.29 47.62,34.78 47.54,34.87 47.54,36.91 45.72,38.73 v31.75,38.73
N$110
  Top 0.25: R24.1 IC2.2
N$111  (via drill 0.35)
  Top 0.25: R25.1 29.21,13.15 29.21,14.61 31.75,17.14 v38.1,17.14 | v42.1,14.61 IC2.15
  Bottom 0.25: v38.1,17.14 38.73,17.14 40.64,15.24 40.64,14.61 v42.1,14.61
N$112
  Top 0.25: IC2.1 R26.1
N$113
  Top 0.25: R27.1 IC2.6
N$114
  Top 0.25: IC2.7 R28.1
N$115
  Top 0.25: R29.1 IC2.4
N$116
  Top 0.25: IC2.9 arc90 43.68,6.95 R30.1
N$117
  Top 0.25: R31.1 IC2.5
